PROGRAM PRG_READ_List_Array
VAR
	fbUA_Connect			: UA_Connect;
	SessionConnectInfo		: ST_UASessionConnectInfo;
	sOpcUA_URL				: STRING(MAX_STRING_LENGTH);
	nConnectionHdl			: DWORD;

	fbUA_GetNamespaceIndex 	: UA_GetNamespaceIndex;
	nNamespaceIndex			: UINT;
	fbUA_NodeGetHandleList	: UA_NodeGetHandleList;
	NodeIDs					: ARRAY [1..nMaxNodeIDsInList] OF ST_UANodeID;
	nNodeHdls				: ARRAY [1..nMaxNodeIDsInList] OF DWORD;

	fbUA_ReadList			: UA_ReadList; 
	stIndexRange			: ARRAY [1..nMaxIndexRange] OF ST_UAIndexRange;
	nIndexRangeCount		: UINT;
	stNodeAddInfo			: ARRAY [1..nMaxNodeIDsInList] OF ST_UANodeAdditionalInfo;
	stReadListDataArrayInt	: ST_ReadListData_Array; // memory block must contain the Data[], NodeErrorIDs[], TimeStamps[] and cbData_R[]
	cbData					: ARRAY [1..nMaxNodeIDsInList] OF UDINT; (* Bytes to be actually Read *)
	cbData_R				: UDINT;
	cbDataTotal				: UDINT; 
	
	fbUA_NodeReleaseHandleList	: UA_NodeReleaseHandleList;

	fbUA_Disconnect		: UA_Disconnect;

	iState		: INT;
	bTest		: BOOL:= TRUE;
	bDone		: BOOL;
	bBusy		: BOOL;
	bError		: BOOL;
	nErrorID	: DWORD;
	
	nNodeIdx	: INT; 
END_VAR


CASE iState OF
0:	(* idle *)
	IF bTest THEN
		bTest		:= FALSE;
		bError		:= FALSE;
		nErrorID	:= 0;

		SessionConnectInfo.tConnectTimeout 		:= T#1M;
		SessionConnectInfo.tSessionTimeout 		:= T#1M;
		SessionConnectInfo.sApplicationName		:= '';
		SessionConnectInfo.eSecurityMode 		:= eUASecurityMsgMode_None;
		SessionConnectInfo.eSecurityPolicyUri 	:= eUASecurityPolicy_None;
		SessionConnectInfo.eTransportProfileUri := eUATransportProfileUri_UATcp;

		iState	:= iState + 1;
	END_IF

1:	(* open UA session *)
	fbUA_Connect(
		Execute				:= TRUE,
		ServerURL			:= sOpcUaServerUrl,
		SessionConnectInfo  := SessionConnectInfo,
		Timeout				:= T#2M,
		ConnectionHdl		=> nConnectionHdl
	);

	IF NOT fbUA_Connect.Busy THEN
		fbUA_Connect(Execute := FALSE);

		IF NOT fbUA_Connect.Error THEN
			(* session open *)
			iState := iState + 1;
		ELSE
			bError			:= TRUE;
			nErrorID		:= fbUA_Connect.ErrorID;
			nConnectionHdl	:= 0;
			iState 			:= 0; (* idle *)
		END_IF
	END_IF


2:	(* GetNS Index *)
	fbUA_GetNamespaceIndex(
		Execute			:= TRUE,
		ConnectionHdl	:= nConnectionHdl,
		NamespaceUri	:= sNamespaceUri,
		NamespaceIndex	=> nNamespaceIndex
	);

	IF NOT fbUA_GetNamespaceIndex.Busy THEN
		fbUA_GetNamespaceIndex(Execute := FALSE);
		IF NOT fbUA_GetNamespaceIndex.Error THEN
			(* session closed *)
			iState 		:= iState + 1; (* idle *)
		ELSE
			bError		:= TRUE;
			nErrorID	:= fbUA_GetNamespaceIndex.ErrorID;
			iState 		:= 6; (* idle *)
		END_IF
	END_IF


3:	(* Get Node Handle *)

	nNodeIdx := 1;
	NodeIDs[nNodeIdx].eIdentifierType := eUAIdentifierType_String;
	NodeIDs[nNodeIdx].nNamespaceIndex := nNamespaceIndex;
	NodeIDs[nNodeIdx].sIdentifier	:= 'MAIN.iArrayIntVar1';
	
	nNodeIdx := nNodeIdx + 1;
	NodeIDs[nNodeIdx].eIdentifierType := eUAIdentifierType_String;
	NodeIDs[nNodeIdx].nNamespaceIndex := nNamespaceIndex;
	NodeIDs[nNodeIdx].sIdentifier	:= 'MAIN.iArrayIntVar2';

	fbUA_NodeGetHandleList(
		Execute			:= TRUE,
		ConnectionHdl	:= nConnectionHdl,
		NodeIDCount 	:= nNodeIdx,
		NodeIDs			:= NodeIDs,
		NodeHdls		=> nNodeHdls
	);

	IF NOT fbUA_NodeGetHandleList.Busy THEN
		fbUA_NodeGetHandleList(Execute := FALSE);

		IF NOT fbUA_NodeGetHandleList.Error THEN
			(* session closed *)
			iState 		:= iState + 1; (* idle *)
		ELSE
			bError		:= TRUE;
			nErrorID	:= fbUA_NodeGetHandleList.ErrorID;
			iState 		:= 6; (* idle *)
		END_IF
	END_IF

	
4: 	(* UA_Read *)
	cbData[1] := SIZEOF(stReadListDataArrayInt.iArrayIntVar1);
	cbData[2] := SIZEOF(stReadListDataArrayInt.iArrayIntVar2);

	cbDataTotal := SIZEOF(stReadListDataArrayInt);
	fbUA_ReadList(
		Execute			:= TRUE,
		ConnectionHdl	:= nConnectionHdl,
		NodeHdlCount	:= nNodeIdx, // 2
		NodeHdls		:= nNodeHdls,
		stNodeAddInfo 	:= stNodeAddInfo,
		pVariable		:= ADR(stReadListDataArrayInt),
		cbData			:= cbData ,
		cbDataTotal		:= cbDataTotal		
		);

	IF NOT fbUA_ReadList.Busy THEN
		fbUA_ReadList( Execute := FALSE, cbData_R => cbData_R);

		IF NOT fbUA_ReadList.Error THEN
			(* session closed *)
			iState 		:= iState + 1; (* idle *)
		ELSE
			bError		:= TRUE;
			nErrorID	:= fbUA_ReadList.ErrorID;
			iState 		:= 6; (* idle *)
		END_IF
	END_IF


5:	(* Release Node Handle *)
	fbUA_NodeReleaseHandleList(
		Execute			:= TRUE,
		ConnectionHdl	:= nConnectionHdl,
		NodeHdlCount	:= nNodeIdx,
		NodeHdls		:= nNodeHdls
	);

	IF NOT fbUA_NodeReleaseHandleList.Busy THEN
		fbUA_NodeReleaseHandleList(Execute := FALSE);

		IF NOT fbUA_NodeReleaseHandleList.Error THEN
			(* session closed *)
			iState 		:= iState + 1; (* idle *)
		ELSE
			bError		:= TRUE;
			nErrorID	:= fbUA_NodeReleaseHandleList.ErrorID;
			iState 		:= 6; (* idle *)
		END_IF
	END_IF


6:	(* close session *)
	fbUA_Disconnect(
		Execute			:= TRUE,
		ConnectionHdl	:= nConnectionHdl
	);

	IF NOT fbUA_Disconnect.Busy THEN
		fbUA_Disconnect(Execute := FALSE);
		bBusy := FALSE;
		IF NOT fbUA_Disconnect.Error THEN
			(* session closed *)
			iState 		:= 0; (* idle *)
			IF NOT bError THEN 
				bDone 	:= TRUE;
			END_IF
		ELSE
			bError			:= TRUE;
			nErrorID		:= fbUA_Disconnect.ErrorID;
			iState 			:= 0; (* idle *)
			nConnectionHdl	:= 0;
		END_IF
	END_IF
END_CASE

END_PROGRAM
